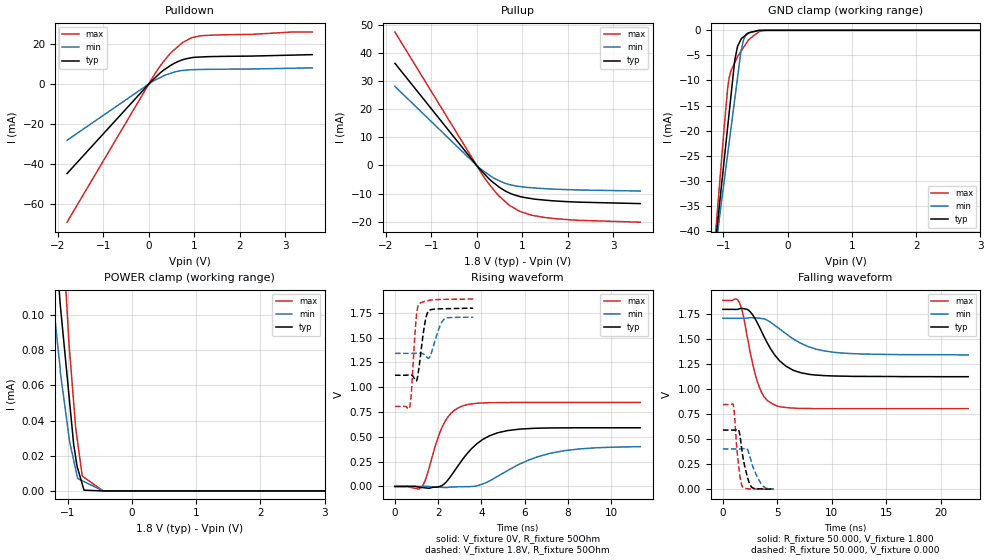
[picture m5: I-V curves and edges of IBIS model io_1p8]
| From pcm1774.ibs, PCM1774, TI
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|   io_1p8 Model
[Model]   io_1p8
Model_type   I/O
Polarity   Non-Inverting
Enable   Active-Low
Vinl = 0.54
Vinh = 1.26
Vmeas = 0.9
Vref = 0.9
Cref = 10pF
Rref = 50
|   typ   min   max
|   (nom PVT)   (fast PVT)   (slow PVT)
C_comp   8.925e-13   8.892e-13   9.027e-13
|ON state : BUFFER OUTPUT TURNED HIGH
|C_comp   8.925e-13   8.892e-13   9.027e-13
|OFF state: BUFFER IN HIGH IMPEDANCE
|C_comp   8.959e-13   8.859e-13   9.027e-13
| Where nom  PVT is Nominal Process, 1.8V, 26C
|   Fast PVT is Strong Process,  1.89V, -40C
|   Slow PVT is Weak Process,   1.71V, 86C
[Model Spec]
|Subparameter   typ   min   max
Vinh   1.26   1.197   1.323
Vinl   0.54   0.513   0.567
[Voltage Range]   1.8   1.71   1.89
|Ambient Temperature   25   85   -40
|Junction Temperature
[Temperature Range]   26   86   -40
[Pullup Reference]   1.8   1.71   1.89
[Pulldown Reference]   0   0   0
[Power Clamp Reference]   1.8   1.71   1.89
[GND Clamp Reference]   0   0   0
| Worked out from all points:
|   slope of the pulldown table from 0 to 0.27 V, typ, clamps not added: 45.5 ohm
|   slope of the pullup table from 0 to 0.27 V, typ, clamps not added: 57 ohm
|   GND clamp passes 1 mA (typ) near -0.66 V on its own axis
|   falling waveform, R_fixture 50.000, V_fixture 1.800: 20-80 % time 2.31ns typ, 3.31ns min, 1.35ns max; typ from 1.8 V to 1.13 V
|   rising waveform, V_fixture 0V, R_fixture 50Ohm: 20-80 % time 1.42ns typ, 2.38ns min, 822ps max; typ from 0 V to 0.592 V
|   rising waveform, V_fixture 1.8V, R_fixture 50Ohm: 20-80 % time 252ps typ, 336ps min, 190ps max; typ from 1.12 V to 1.8 V
|   falling waveform, R_fixture 50.000, V_fixture 0.000: 20-80 % time 613ps typ, 864ps min, 408ps max; typ from 0.592 V to 0.001 V
[Pulldown]
|   Voltage   I(typ)   I(min)   I(max)
-1.8V     -44.89mA   -28.22mA   -69.28mA
21.6mV    579.7uA    344.4uA    909.9uA
178.8mV   4.002mA    2.439mA    6.681mA
333mV     7.079mA    4.211mA    11.46mA
486.9mV   9.446mA    5.428mA    15.66mA
749.6mV   12.2mA     6.806mA    20.89mA
948.1mV   13.24mA    7.174mA    23.24mA
1.177V    13.59mA    7.312mA    24.25mA
2.254V    14.01mA    7.532mA    24.88mA
3.127V    14.48mA    7.9mA      26.04mA
3.6V      14.73mA    8.102mA    26.04mA
[GND Clamp]
|   Voltage   I(typ)   I(min)   I(max)
-1.8V     -127.5mA   -112.9mA   -149.8mA
-1.097V   -39.15mA   -40.96mA   -36.35mA
-1.051V   -33.41mA   -36.28mA   -29.18mA
-934.4mV  -19.27mA   -24.66mA   -11.54mA
-909.8mV  -16.3mA    -22.23mA   -9.42mA
-826.2mV  -6.18mA    -13.94mA   -6.489mA
-781.2mV  -3.226mA   -9.481mA   -5.245mA
-727.8mV  -1.827mA   -4.253mA   -4.203mA
-688.5mV  -1.308mA   -1.925mA   -3.439mA
-640.6mV  -839.8uA   -651.7uA   -2.509mA
-346.6mV  -77.46nA   0A         -18.33uA
3.6V      0A         0A         0A
[Pullup]
|   Voltage   I(typ)   I(min)   I(max)
-1.8V     36.41mA    28.18mA    47.55mA
630uV     -47.78uA   -30.98uA   -67.59uA
103.2mV   -1.872mA   -1.449mA   -2.732mA
257.4mV   -4.547mA   -3.21mA    -6.347mA
409.4mV   -6.64mA    -4.726mA   -9.438mA
563.4mV   -8.455mA   -5.935mA   -11.94mA
715.6mV   -9.781mA   -6.8mA     -14.16mA
953.7mV   -11.08mA   -7.491mA   -16.4mA
1.177V    -11.74mA   -7.897mA   -17.59mA
1.481V    -12.32mA   -8.247mA   -18.5mA
2.252V    -13.07mA   -8.733mA   -19.55mA
3.6V      -13.58mA   -9.102mA   -20.21mA
[POWER Clamp]
|   Voltage   I(typ)   I(min)   I(max)
-1.8V     771.6uA    463.1uA    733.6uA
-1.398V   249.9uA    166.6uA    369.5uA
-1.131V   114.1uA    75.02uA    179.2uA
-1.113V   105.2uA    67.24uA    167.7uA
-979.7mV  54.61uA    30.93uA    84.7uA
-907.2mV  27uA       17.69uA    50.94uA
-873.9mV  18.94uA    12.1uA     35.58uA
-844.1mV  12.87uA    7.105uA    27.65uA
-771.8mV  3.79uA     5.805uA    8.415uA
-745.2mV  443.1nA    5.326uA    7.721uA
-448.6mV  0A         0A         0A
3.6V      0A         0A         0A
[Ramp]
R_load = 50
|   typ   min   max
dV/dt_r   0.355122/1.42513e-09   0.241989/2.40603e-09   0.508279/8.22296e-10
dV/dt_f   0.405466/2.32411e-09   0.216865/3.35537e-09   0.650403/1.35003e-09
[Falling Waveform]
R_fixture = 50.000
V_fixture = 1.800
V_fixture_min = 1.710
V_fixture_max = 1.890
C_fixture = 0.000
|   Time   V(typ)   V(min)   V(max)
0s        1.8V       1.71V      1.89V
1.51ns    1.806V     1.71V      1.869V
1.891ns   1.807V     1.71V      1.73V
2.399ns   1.788V     1.716V     1.434V
3.182ns   1.661V     1.713V     1.072V
3.796ns   1.524V     1.704V     924mV
4.888ns   1.327V     1.63V      837mV
6.488ns   1.189V     1.503V     812mV
9.96ns    1.134V     1.373V     806mV
22.54ns   1.126V     1.344V     806mV
[Rising Waveform]
V_fixture = 0V
V_fixture_min = 0V
V_fixture_max = 0V
R_fixture = 50Ohm
|   Time   V(typ)   V(min)   V(max)
0s        333pV      635.1pV    252.7pV
1.245ns   -10.38mV   575.9uV    -3.662mV
2.269ns   23.73mV    -10.16mV   636.6mV
2.707ns   142.2mV    -4.606mV   761mV
3.182ns   288.3mV    -2.653mV   815.8mV
4.059ns   473.9mV    25.56mV    842.2mV
5.212ns   563.6mV    160.7mV    846.3mV
6.578ns   587.2mV    297.8mV    846.9mV
7.845ns   590.7mV    361.1mV    846.9mV
11.35ns   591.6mV    400.7mV    847mV
[Rising Waveform]
V_fixture = 1.8V
V_fixture_min = 1.71V
V_fixture_max = 1.89V
R_fixture = 50Ohm
|   Time   V(typ)   V(min)   V(max)
0s        1.121V     1.342V     806mV
691.3ps   1.125V     1.342V     809.9mV
760ps     1.124V     1.342V     948.2mV
969.8ps   1.064V     1.343V     1.666V
1.037ns   1.094V     1.344V     1.79V
1.123ns   1.217V     1.345V     1.842V
1.369ns   1.629V     1.326V     1.865V
1.543ns   1.767V     1.292V     1.875V
2.264ns   1.792V     1.685V     1.886V
3.62ns    1.797V     1.707V     1.889V
[Falling Waveform]
R_fixture = 50.000
V_fixture = 0.000
V_fixture_min = 0.000
V_fixture_max = 0.000
C_fixture = 0.000
|   Time   V(typ)   V(min)   V(max)
0s        591.9mV    403.3mV    847.1mV
969.7ps   591.5mV    403.1mV    840.4mV
1.286ns   596.4mV    403mV      406.3mV
1.449ns   591.8mV    402.9mV    236.3mV
1.631ns   489.4mV    402.9mV    87.08mV
1.81ns    342.8mV    404.4mV    23.07mV
2.264ns   119mV      397.6mV    4.526mV
2.639ns   20.27mV    265.4mV    2.17mV
3.62ns    2.505mV    39.38mV    1.115mV
4.666ns   1.144mV    3.518mV    284uV
